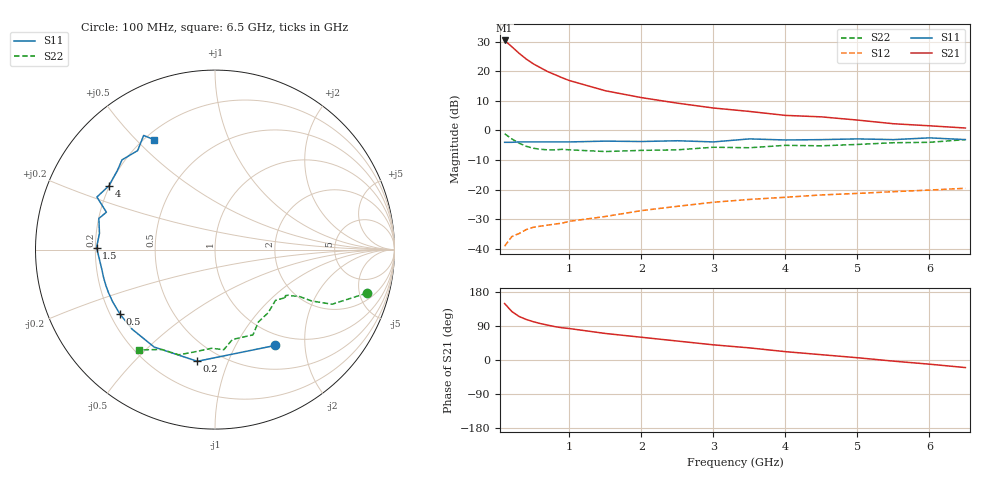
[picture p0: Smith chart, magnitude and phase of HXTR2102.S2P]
! HXTR-2102 Common Emitter
! Vce=15V  Ic=25mA
# ghz s ma r 50
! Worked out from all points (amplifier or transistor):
!   21 points, 100 MHz to 6.5 GHz, reference 50 ohm
!   highest |S21| = 30.5 dB at 100 MHz (marker M1)
!   |S21| within 3 dB of that: start of sweep to 240.2 MHz
!   unconditionally stable (mu >= 1): 1.083 GHz to 3.407 GHz; 3.81 GHz to 4.304 GHz
!   at 400 MHz: K = 0.54, MSG = 28.9 dB, |S12| = -33.6 dB
!   at 1.5 GHz: K = 1.19, MAG = 18.6 dB, |S12| = -29.1 dB
!   at 6.5 GHz: K = 0.71, MSG = 10.2 dB, |S12| = -19.6 dB
!   S11 on the Smith chart (normalised r, x): 100 MHz: 0.83, -1.47; 200 MHz: 0.38, -0.78; 500 MHz: 0.24, -0.29; 1.5 GHz: 0.20, +0.01; 4 GHz: 0.20, +0.27; 6.5 GHz: 0.24, +0.56
0.1  0.63 -58.0  33.4 149.0  0.011 62.0  0.88 -16.0
0.2  0.63 -99.0  26.2 128.0  0.016 49.0  0.72 -25.0
0.3  0.64 -122.0  20.3 115.0  0.018 45.0  0.61 -28.0
0.4  0.64 -136.0  16.2 107.0  0.021 42.0  0.54 -29.0
0.5  0.64 -146.0  13.4 101.0  0.023 42.0  0.5 -31.0
0.6  0.64 -153.0  11.5 96.0  0.024 43.0  0.48 -32.0
0.7  0.64 -158.0  9.9 92.0  0.025 43.0  0.47 -33.0
0.8  0.64 -162.0  8.8 88.0  0.026 45.0  0.47 -34.0
0.9  0.64 -166.0  7.8 85.0  0.027 44.0  0.48 -34.0
1  0.64 -170.0  7 83.0  0.029 46.0  0.47 -35.0
1.5  0.66 179.0  4.7 70.0  0.035 49.0  0.44 -40.0
2  0.65 172.0  3.6 60.0  0.044 53.0  0.46 -50.0
2.5  0.67 165.0  2.9 50.0  0.052 55.0  0.47 -59.0
3  0.64 161.0  2.4 40.0  0.061 57.0  0.52 -66.0
3.5  0.72 156.0  2.1 32.0  0.068 53.0  0.51 -79.0
4  0.69 149.0  1.8 22.0  0.074 48.0  0.56 -85.0
4.5  0.7 141.0  1.7 14.0  0.081 44.0  0.55 -92.0
5  0.72 136.0  1.5 6.0  0.086 39.0  0.58 -101.0
5.5  0.7 128.0  1.3 -3.0  0.092 34.0  0.62 -109.0
6  0.75 122.0  1.2 -11.0  0.098 30.0  0.63 -118.0
6.5  0.7 119.0  1.1 -20.0  0.105 26.0  0.7 -127.0
